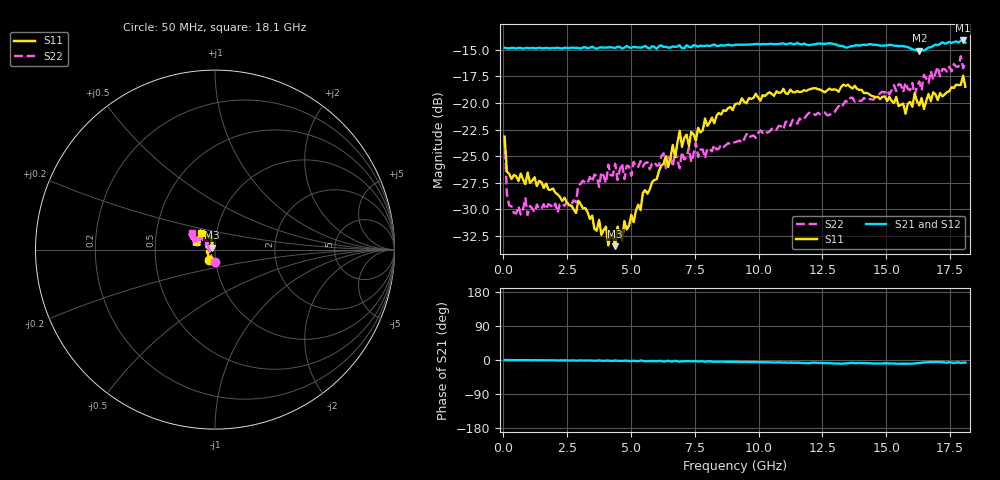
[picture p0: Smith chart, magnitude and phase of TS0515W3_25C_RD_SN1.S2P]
! Network Analyzer HP8720D.06.14 Serial No. US36140669
! 17 Jun 2005  08:36:41
! Frequency  S11  S21  S12  S22
# HZ  S  DB R 50
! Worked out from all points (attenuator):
!   201 points, 50 MHz to 18.1 GHz, reference 50 ohm
!   highest |S21| = -14.12 dB at 18.01 GHz (marker M1); lowest = -15.1 dB at 16.3 GHz (marker M2)
!   lowest |S11| = -33.5 dB at 4.382 GHz (marker M3), VSWR 1.04, Z = 48.1 + j0.949 ohm
!   |S11| at or under -10 dB: start of sweep to end of sweep
!   |S22| runs from -30.6 to -15.6 dB; largest |S21 - S12| = 0.0055
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5e7  -23.17 -119.9  -14.80 -0.1  -14.80 0.0  -23.32 -89.8
1.4025e8  -26.45 -143.1  -14.84 -0.2  -14.85 -0.1  -28.58 -129.4
4.11e8  -26.78 -163.1  -14.82 -0.2  -14.84 -0.2  -30.33 -158.9
2.12575e9  -28.61 -165.8  -14.80 -1.2  -14.83 -1.1  -30.32 162.6
3.1185e9  -29.92 -170.9  -14.78 -1.5  -14.81 -1.5  -27.31 168.2
4.382e9  -33.48 152.3  -14.83 -1.5  -14.75 -2.1  -25.72 163.4
4.47225e9  -31.63 144.5  -14.71 -2.0  -14.76 -1.6  -27.25 166.4
4.65275e9  -32.92 136.9  -14.89 -2.2  -14.75 -2.0  -25.69 166.1
4.743e9  -31.12 139.2  -14.79 -2.0  -14.81 -1.9  -27.17 161.4
6.09675e9  -26.40 110.5  -14.65 -2.5  -14.61 -2.6  -25.87 154.6
6.7285e9  -25.12 112.6  -14.73 -2.2  -14.81 -2.9  -24.55 148.6
6.909e9  -22.62 110.4  -14.57 -4.3  -14.69 -3.9  -26.13 143.2
7.27e9  -24.06 107.4  -14.72 -2.9  -14.73 -3.8  -24.19 145.4
7.36025e9  -22.71 104.9  -14.77 -3.6  -14.71 -3.1  -25.58 148.1
7.54075e9  -23.55 106.3  -14.62 -3.0  -14.53 -4.1  -23.77 147.7
7.90175e9  -21.45 114.4  -14.64 -4.5  -14.61 -3.9  -25.20 140.6
9.075e9  -20.12 125.0  -14.53 -4.8  -14.52 -4.7  -23.71 137.0
1.21435e10  -18.62 157.1  -14.49 -6.8  -14.48 -7.0  -21.03 138.7
1.512175e10  -19.42 162.4  -14.52 -9.1  -14.50 -8.7  -19.20 151.6
1.6295e10  -20.23 150.4  -15.09 -8.2  -15.00 -8.3  -17.98 159.3
1.800975e10  -17.43 127.5  -14.12 -6.9  -14.25 -6.7  -16.73 151.0
1.81e10  -18.48 129.3  -14.33 -6.8  -14.37 -8.2  -16.17 143.9
